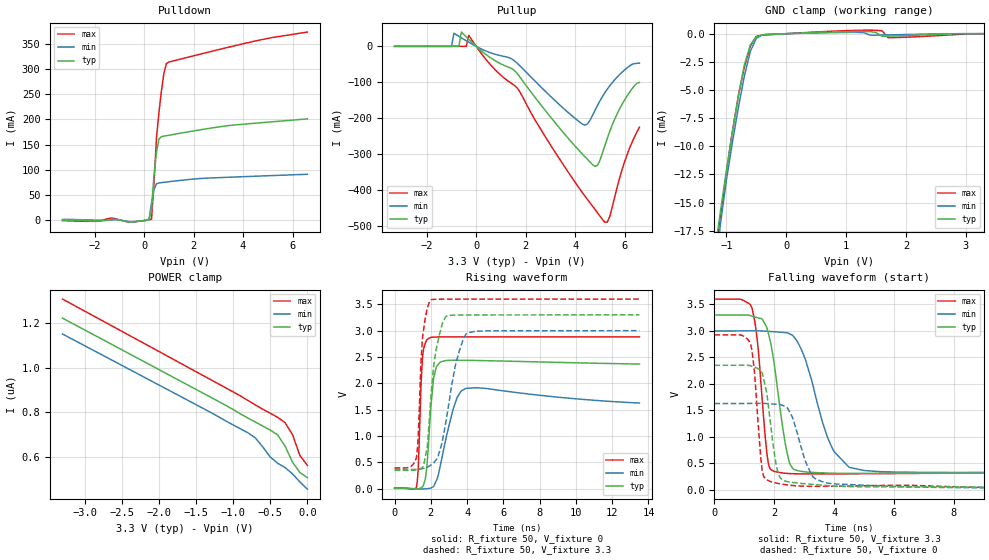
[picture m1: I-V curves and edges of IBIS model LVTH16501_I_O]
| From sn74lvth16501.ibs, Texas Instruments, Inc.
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|************* LVTH16501 OUTPUT (3.3 V) MODEL**************
[Model]   LVTH16501_I_O
Model_type  I/O
Polarity   Non-Inverting
Enable   Active-Low
Vinl = 0.8V
Vinh = 2.0V
Vmeas = 1.5V
Cref = 50pF
Rref = 500
Vref = 0
| variable   typ   min   max
C_comp   12p   NA   NA
[Temperature Range]   50   100   0
[Voltage range]   3.3   3   3.6
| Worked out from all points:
|   slope of the pulldown table from 0 to 0.495 V, typ, clamps not added: 3.73 ohm
|   slope of the pullup table from 0 to 0.495 V, typ, clamps not added: 17.8 ohm
|   GND clamp passes 1 mA (typ) near -0.60 V on its own axis
|   rising waveform, R_fixture 50, V_fixture 0: 20-80 % time 302ps typ, 622ps min, 182ps max; typ from 0.006 V to 2.37 V
|   falling waveform, R_fixture 50, V_fixture 3.3: 20-80 % time 451ps typ, 837ps min, 293ps max; typ from 3.3 V to 0.325 V
|   rising waveform, R_fixture 50, V_fixture 3.3: 20-80 % time 496ps typ, 832ps min, 268ps max; typ from 0.347 V to 3.3 V
|   falling waveform, R_fixture 50, V_fixture 0: 20-80 % time 332ps typ, 553ps min, 236ps max; typ from 2.35 V to 0.028 V
|Process range|   weak   strong
[Pullup]
|   50C:3.3V:   100C:3V:weak   0C:3.6V:strong
|   Voltage   I(typ)   I(min)   I(max)
-3.3V     70.97uA    42.59uA    121.4uA
-700mV    57.28uA    27.84mA    109.7uA
-600mV    39.72mA    23.68mA    108.8uA
-400mV    26.25mA    15.53mA    64.69uA
-300mV    19.6mA     11.54mA    30.71mA
1.6V      -70.77mA   -43.37mA   -111.6mA
4.3V      -299.8mA   -216.6mA   -407.2mA
4.8V      -333.6mA   -178.4mA   -453mA
5.2V      -276.4mA   -129.2mA   -488.9mA
5.4V      -236.5mA   -109.7mA   -473mA
5.9V      -160.8mA   -71.81mA   -342.3mA
6.6V      -100.4mA   -46.63mA   -224.8mA
[Pulldown]
|   50C:3.3V:   100C:3V:weak   0C:3.6V:strong
|   Voltage   I(typ)   I(min)   I(max)
-3.3V     332.6uA    1.888mA    -241uA
-1.3V     2.202mA    1.028mA    4.704mA
100mV     446.7uA    438.3uA    436.3uA
200mV     1.158mA    2.926mA    1.112mA
300mV     23.17mA    35.42mA    2.898mA
400mV     90.36mA    61.52mA    74.52mA
500mV     134.9mA    72.51mA    164mA
600mV     161.2mA    74.23mA    213.6mA
800mV     166.9mA    75.5mA     291.2mA
900mV     167.8mA    76.1mA     310.4mA
4.3V      191.7mA    87.22mA    353mA
6.6V      201mA      91.47mA    372.8mA
[GND Clamp]
|   50C:3.3V:   100C:3V:weak   0C:3.6V:strong
|   Voltage   I(typ)   I(min)   I(max)
-3.3V     -709.5mA   -633.2mA   -786.3mA
-1.2V     -19.66mA   -22.36mA   -20.1mA
-1.1V     -15.79mA   -16.9mA    -16.14mA
-1V       -12.17mA   -13.01mA   -12.28mA
-800mV    -5.573mA   -6.561mA   -5.493mA
-700mV    -2.789mA   -3.769mA   -2.954mA
-600mV    -993.3uA   -1.56mA    -1.088mA
-500mV    -281.9uA   -413.4uA   -233.2uA
1.3V      192.9uA    85.4uA     308.7uA
1.6V      -219.5uA   -116.3uA   263uA
1.7V      -212.3uA   -107uA     -348.4uA
3.3V      505.9nA    550.9nA    495.1nA
[POWER Clamp]
|   50C:3.3V:   100C:3V:weak   0C:3.6V:strong
|   Voltage   I(typ)   I(min)   I(max)
-3.3V     1.222uA    1.15uA     1.307uA
-1.1V     830.2nA    760.3nA    908.7nA
-800mV    772.9nA    706.8nA    852nA
-700mV    754.9nA    683.7nA    831.8nA
-600mV    737.1nA    643.4nA    812.7nA
-500mV    719.2nA    598.1nA    794.5nA
-400mV    697.2nA    570.3nA    776.2nA
-300mV    647nA      550.9nA    752.5nA
-200mV    575.5nA    522.6nA    698.8nA
-100mV    528.5nA    486.2nA    604.6nA
0V        505.9nA    453.9nA    560.9nA
[ramp]
| variable   typ   min   max
dV/dt_r   1.4671E+00/3.4444E-10  1.1330E+00/8.9888E-10  1.7349E+00/1.8194E-10
dV/dt_f   1.7932E+00/4.4847E-10  1.6021E+00/8.4243E-10  1.9787E+00/2.9155E-10
[Rising Waveform]
R_fixture = 50
V_fixture = 0
V_fixture_min = 0
V_fixture_max = 0
C_fixture = 0
L_fixture = 0
|   50C:3.3V:   100C:3V:weak   0C:3.6V:strong
|   Time   V(typ)   V(min)   V(max)
0s        5.759mV    4.174mV    7.896mV
1.2ns     -10.07mV   -4.269mV   13.58mV
1.3ns     -3.928mV   -6.471mV   355.3mV
1.55ns    38.9mV     -7.464mV   2.528V
1.75ns    323.7mV    -3.678mV   2.813V
1.9ns     1.025V     3.282mV    2.857V
2.3ns     2.311V     151.2mV    2.879V
3.25ns    2.437V     1.532V     2.882V
3.9ns     2.436V     1.899V     2.882V
13.5ns    2.365V     1.625V     2.882V
[Falling Waveform]
R_fixture = 50
V_fixture = 3.3
V_fixture_min = 3
V_fixture_max = 3.6
C_fixture = 0
L_fixture = 0
|   50C:3.3V:   100C:3V:weak   0C:3.6V:strong
|   Time   V(typ)   V(min)   V(max)
0s        3.3V       3V         3.6V
1.25ns    3.28V      3.001V     3.438V
1.45ns    3.248V     3.001V     2.731V
1.75ns    3.066V     2.994V     700mV
1.95ns    2.55V      2.986V     363.5mV
2.4ns     773.6mV    2.968V     314.4mV
2.65ns    387.7mV    2.892V     306.7mV
3.8ns     318.9mV    961.5mV    304.3mV
4.5ns     313.7mV    427.8mV    306.3mV
13.5ns    325.1mV    342.4mV    333.3mV
[Rising Waveform]
R_fixture = 50
V_fixture = 3.3
V_fixture_min = 3
V_fixture_max = 3.6
C_fixture = 0
L_fixture = 0
|   50C:3.3V:   100C:3V:weak   0C:3.6V:strong
|   Time   V(typ)   V(min)   V(max)
0s        347.3mV    361.4mV    391mV
1.2ns     356.1mV    364.6mV    583.1mV
1.3ns     364.6mV    367.3mV    962.4mV
1.55ns    400.5mV    380.4mV    2.893V
1.8ns     782.5mV    406.9mV    3.412V
2ns       1.735V     445.8mV    3.585V
2.65ns    3.154V     936.6mV    3.598V
3.35ns    3.295V     2.338V     3.599V
4ns       3.297V     2.956V     3.6V
13.5ns    3.3V       3V         3.6V
[Falling Waveform]
R_fixture = 50
V_fixture = 0
V_fixture_min = 0
V_fixture_max = 0
L_fixture = 0
C_fixture = 0
|   50C:3.3V:   100C:3V:weak   0C:3.6V:strong
|   Time   V(typ)   V(min)   V(max)
0s        2.352V     1.63V      2.925V
1.2ns     2.344V     1.633V     2.764V
1.35ns    2.316V     1.634V     2.146V
1.6ns     2.202V     1.635V     342.7mV
1.85ns    1.363V     1.627V     163.5mV
2.2ns     229.4mV    1.609V     116.5mV
2.6ns     143.3mV    1.379V     85.61mV
3.25ns    107.2mV    280.2mV    69.38mV
3.8ns     82mV       128mV      69.78mV
13.5ns    28.15mV    30.04mV    15.94mV
